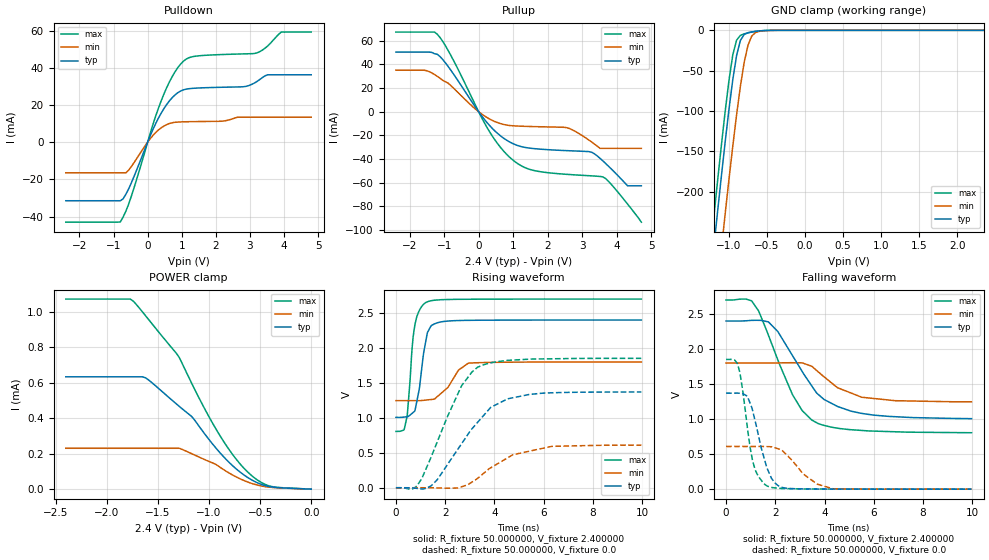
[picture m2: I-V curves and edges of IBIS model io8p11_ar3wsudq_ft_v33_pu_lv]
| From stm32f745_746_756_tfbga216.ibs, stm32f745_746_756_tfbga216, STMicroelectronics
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|   Model io8p11_ar3wsudq_ft_v33_pu_lv
[Model]  io8p11_ar3wsudq_ft_v33_pu_lv
Model_type I/O
Polarity   Non-Inverting
Enable   Active-Low
Vinl =   0.720000V
Vinh =   1.680000V
Vmeas =  1.200000V
Cref =   30.000000pF
Rref =   100.000000M
Vref =   0.0V
C_comp   3.742400pF   3.690400pF   3.817400pF
[Temperature Range]   25.000000   0.125000k   -40.000000
[Pullup Reference]   2.400000V   1.800000V   2.700000V
[Pulldown Reference]   0.0V   0.0V   0.0V
[POWER Clamp Reference]   2.400000V   1.800000V   2.700000V
[GND Clamp Reference]   0.0V   0.0V   0.0V
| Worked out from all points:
|   slope of the pulldown table from 0 to 0.36 V, typ, clamps not added: 25 ohm
|   slope of the pullup table from 0 to 0.36 V, typ, clamps not added: 27.7 ohm
|   GND clamp passes 1 mA (typ) near -0.62 V on its own axis
|   rising waveform, R_fixture 50.000000, V_fixture 2.400000: 20-80 % time 349ps typ, 709ps min, 272ps max; typ from 1.01 V to 2.4 V
|   rising waveform, R_fixture 50.000000, V_fixture 0.0: 20-80 % time 1.73ns typ, 1.69ns min, 1.37ns max; typ from 0.001 V to 1.37 V
|   falling waveform, R_fixture 50.000000, V_fixture 2.400000: 20-80 % time 1.64ns typ, 1.49ns min, 1.4ns max; typ from 2.4 V to 1.01 V
|   falling waveform, R_fixture 50.000000, V_fixture 0.0: 20-80 % time 600ps typ, 1.04ns min, 461ps max; typ from 1.37 V to 0.001 V
[Pulldown]
|Voltage   I(typ)   I(min)   I(max)
-2.4V     -31.47mA   -16.45mA   -43.01mA
-800mV    -31.47mA   -16.45mA   -42.85mA
-480mV    -21.98mA   -13.17mA   -29.21mA
80mV      3.63mA     1.966mA    5.014mA
480mV     18.16mA    8.738mA    26.02mA
800mV     25.38mA    10.72mA    37.77mA
1.12V     28.53mA    11.02mA    44.6mA
2.8V      29.84mA    13.47mA    47.53mA
3.2V      32.6mA     13.47mA    48.03mA
3.52V     36.3mA     13.47mA    51.75mA
3.92V     36.3mA     13.47mA    59.27mA
4.8V      36.3mA     13.47mA    59.27mA
[Pullup]
|Voltage   I(typ)   I(min)   I(max)
-2.4V     50.37mA    35.09mA    67.24mA
-1.52V    50.37mA    34.75mA    67.24mA
-1.2V     48.49mA    29.88mA    65.43mA
-800mV    34.76mA    21.92mA    47.2mA
320mV     -11.75mA   -6.207mA   -17.08mA
1.04V     -27.53mA   -11.97mA   -41.91mA
1.6V      -31.13mA   -12.57mA   -49.63mA
2.56V     -32.88mA   -13.52mA   -52.9mA
3.28V     -34.25mA   -25.62mA   -54.17mA
3.6V      -41.44mA   -30.94mA   -55.02mA
4.32V     -62.6mA    -30.94mA   -77.97mA
4.72V     -62.6mA    -30.94mA   -93.3mA
[GND_clamp]
|Voltage   I(typ)   I(min)   I(max)
-2.4V     -1.437A    -1.518A    -1.41A
-1.25V    -315.9mA   -407.2mA   -278.2mA
-1.2V     -270.1mA   -361.3mA   -232.1mA
-1.15V    -225mA     -316mA     -186.8mA
-1.1V     -180.9mA   -271.3mA   -142.7mA
-1.05V    -138.2mA   -227.5mA   -100.5mA
-950mV    -61.14mA   -143.6mA   -30.43mA
-900mV    -31.23mA   -104.7mA   -12.14mA
-850mV    -12.49mA   -69.4mA    -6.221mA
-750mV    -2.898mA   -18.35mA   -3.18mA
-600mV    -750.2uA   -1.218mA   -738.3uA
2.35V     0A         0A         0A
[POWER_clamp]
|Voltage   I(typ)   I(min)   I(max)
-2.4V     634.4uA    230.9uA    1.073mA
-1.77V    634.4uA    230.9uA    1.073mA
-1.74V    634.4uA    230.9uA    1.062mA
-1.62V    628.7uA    230.9uA    979.3uA
-1.29V    467.4uA    230.9uA    743.1uA
-1.17V    410.9uA    200.6uA    599.2uA
-930mV    230.8uA    139uA      338.2uA
-780mV    138.4uA    83.46uA    204.6uA
-660mV    81.05uA    49.28uA    119.5uA
-540mV    39.7uA     25.07uA    57.27uA
-420mV    15.59uA    11.9uA     19.92uA
0V        0A         0A         0A
[Ramp]
| variable   typ   min   max
dV/dt_r  0.82159/1.73181n   0.36998/1.76752n   1.11113/1.36719n
dV/dt_f  0.83274/1.63962n   0.33186/1.49437n   1.13522/1.40094n
R_load = 50.000000
[Rising Waveform]
R_fixture= 50.000000
V_fixture= 2.400000
V_fixture_min= 1.800000
V_fixture_max= 2.700000
|time   V(typ)   V(min)   V(max)
0s        1.007V     1.247V     806mV
320.3ps   1.011V     1.247V     825.7mV
460.5ps   1.017V     1.247V     1.038V
660.7ps   1.066V     1.247V     2.013V
760.8ps   1.096V     1.247V     2.311V
961ps     1.442V     1.247V     2.543V
1.221ns   2.111V     1.255V     2.652V
1.562ns   2.344V     1.268V     2.683V
2.943ns   2.395V     1.783V     2.697V
9.97ns    2.4V       1.8V       2.7V
[Rising Waveform]
R_fixture= 50.000000
V_fixture= 0.0
V_fixture_min= 0.0
V_fixture_max= 0.0
|time   V(typ)   V(min)   V(max)
0s        958.2uV    875.1uV    1.134mV
860.9ps   -9.184mV   900.2uV    30.73mV
1.261ns   -2.65mV    442uV      302.6mV
1.682ns   116.8mV    -1.617mV   659.7mV
2.663ns   628.1mV    14.18mV    1.457V
3.323ns   938.4mV    136.2mV    1.726V
3.864ns   1.153V     289mV      1.788V
5.405ns   1.335V     522.5mV    1.84V
6.346ns   1.359V     593.1mV    1.846V
9.97ns    1.371V     610.3mV    1.852V
[Falling Waveform]
R_fixture= 50.000000
V_fixture= 2.400000
V_fixture_min= 1.800000
V_fixture_max= 2.700000
|time   V(typ)   V(min)   V(max)
0s        2.4V       1.8V       2.7V
1.041ns   2.409V     1.8V       2.687V
1.321ns   2.41V      1.8V       2.544V
1.722ns   2.387V     1.8V       2.197V
2.703ns   1.904V     1.805V     1.347V
3.103ns   1.674V     1.802V     1.118V
3.724ns   1.359V     1.681V     940.4mV
4.525ns   1.182V     1.449V     870.9mV
5.506ns   1.082V     1.313V     838.8mV
9.97ns    1.007V     1.247V     806mV
[Falling Waveform]
R_fixture= 50.000000
V_fixture= 0.0
V_fixture_min= 0.0
V_fixture_max= 0.0
|time   V(typ)   V(min)   V(max)
0s        1.371V     610.3mV    1.852V
460.5ps   1.371V     610.2mV    1.795V
660.7ps   1.367V     610.1mV    1.446V
860.9ps   1.327V     610mV      895.8mV
1.181ns   974.7mV    609.9mV    279.7mV
1.682ns   287.1mV    608mV      43.83mV
2.262ns   27.65mV    559.1mV    10.65mV
3.143ns   4.788mV    215.5mV    4.163mV
4.344ns   2.361mV    6.359mV    2.134mV
9.97ns    958.2uV    875.1uV    1.134mV
